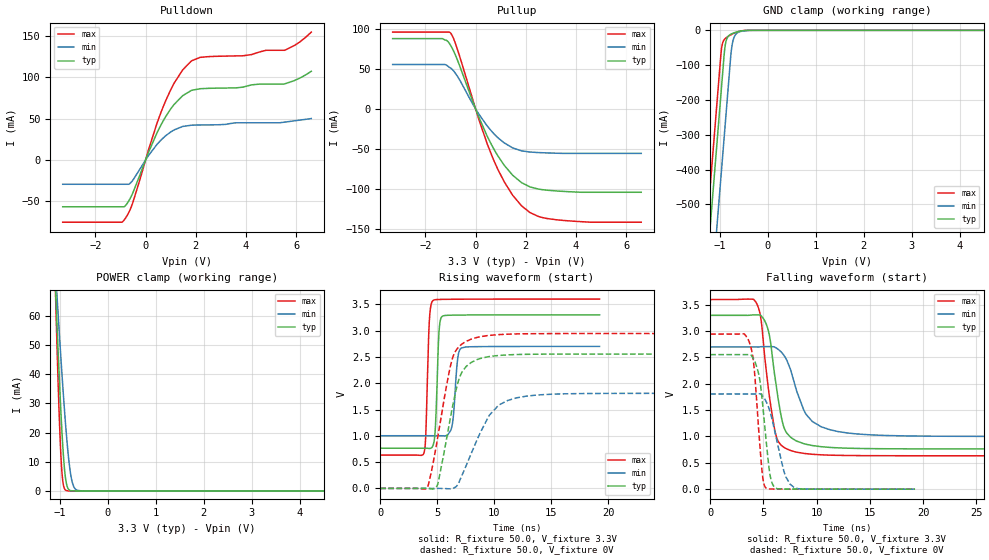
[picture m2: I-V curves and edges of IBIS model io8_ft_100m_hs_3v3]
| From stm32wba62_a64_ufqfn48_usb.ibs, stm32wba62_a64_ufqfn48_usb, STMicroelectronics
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[Model]   io8_ft_100m_hs_3v3
Model_type I/O
Polarity   Non-Inverting
Enable   Active-Low
| CAP_THRESHOLD on pad IOFT is "UDTCAPC" :
| Rising=30.0% of vddiom   Falling=70.0% of vddiom
| C_comp min and max val. don't necessarily correlate with the min and max pvt
| but are the smallest and greatest pad capacitance found.
| var   typ   min   max
C_comp   3.79770pF  3.69238pF  3.85115pF
|C_comp_pullup   2.35247pF  2.17461pF  2.43366pF
|C_comp_pulldown   1.44523pF  1.51776pF  1.41750pF
Vinl = 1.35V
Vinh = 1.8V
Vmeas = 1.65V   | Reference voltage for timing measurements
Cref  = 50.0pF   | Timing specification test load capacitance value
Rref  = 1.0MOhm   | Timing specification test load resistance value
Vref  = 1.815V   | Timing specification test load voltage
[Model Spec]
| TIME_THRESHOLD on pin ZIV11 is "CMOS" :
| Rising=50.0% of vdd   Falling=50.0% of vdd
Vinl 1.29050V 1.08050V 1.37650V
Vinh 1.79850V 1.52050V 1.90250V
| variable   typ   min   max
[Temperature Range] 25.0 140.0 -40.0
| variable   typ   min   max
[Voltage Range] 3.3V 2.7V 3.6V
| variable   typ   min   max
[POWER Clamp Reference] 3.3V 2.7V 3.6V
| variable   typ   min   max
[GND Clamp Reference] 0V 0V 0V
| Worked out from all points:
|   slope of the pulldown table from 0 to 0.495 V, typ, clamps not added: 14 ohm
|   slope of the pullup table from 0 to 0.495 V, typ, clamps not added: 13.8 ohm
|   GND clamp passes 1 mA (typ) near -0.51 V on its own axis
|   POWER clamp passes 1 mA (typ) near -0.83 V on its own axis
|   rising waveform, R_fixture 50.0, V_fixture 3.3V: 20-80 % time 250ps typ, 341ps min, 242ps max; typ from 0.764 V to 3.3 V
|   falling waveform, R_fixture 50.0, V_fixture 3.3V: 20-80 % time 1.12ns typ, 1.98ns min, 1.08ns max; typ from 3.3 V to 0.764 V
|   rising waveform, R_fixture 50.0, V_fixture 0V: 20-80 % time 1.41ns typ, 2.41ns min, 1.46ns max; typ from 0 V to 2.55 V
|   falling waveform, R_fixture 50.0, V_fixture 0V: 20-80 % time 784ps typ, 1.24ns min, 661ps max; typ from 2.55 V to 0 V
[POWER Clamp]
-3.3V     1.123A     753mA      1.645A
-1.09V    69.42mA    75.17mA    67.14mA
-1.08V    65.31mA    72.42mA    61.23mA
-1.06V    57.23mA    66.98mA    49.77mA
-1.01V    38.06mA    53.68mA    24.29mA
-970mV    24.36mA    43.46mA    9.575mA
-930mV    13.06mA    33.74mA    2.352mA
-870mV    3.065mA    20.56mA    165.9uA
-810mV    418.4uA    10.06mA    10.3uA
-760mV    69.41uA    4.321mA    1.009uA
-630mV    611.5nA    197uA      2.727nA
6.6V      0A         0A         0A
[GND Clamp]
-3.3V     -4.134A    -4.372A    -4.018A
-1.59V    -1.227A    -1.465A    -1.111A
-1.25V    -648.9mA   -886.9mA   -533mA
-980mV    -189.9mA   -427.9mA   -74mA
-960mV    -155.9mA   -393.9mA   -48.8mA
-910mV    -70.86mA   -308.9mA   -27.2mA
-880mV    -37.23mA   -257.9mA   -22.76mA
-770mV    -11.28mA   -71.59mA   -12.95mA
-730mV    -8.709mA   -32.74mA   -10.07mA
-630mV    -4.122mA   -6.943mA   -4.354mA
-370mV    -42.68uA   -212.2uA   -13.03uA
6.6V      2.311nA    506.4nA    1.057nA
| variable   typ   min   max
[Pullup Reference] 3.3V 2.7V 3.6V
| variable   typ   min   max
[Pulldown Reference] 0V 0V 0V
[Pullup]
-3.3V     87.39mA    55.15mA    95.56mA
-1.32V    87.39mA    55.15mA    95.56mA
-990mV    78.89mA    50.68mA    94.2mA
-710mV    59.88mA    39.92mA    72.92mA
120mV     -9.566mA   -6.09mA    -12.19mA
460mV     -33.83mA   -21.24mA   -43.26mA
800mV     -54.04mA   -33.36mA   -69.41mA
1.48V     -82.86mA   -48.82mA   -107.8mA
2.17V     -97.42mA   -53.93mA   -129.4mA
2.7V      -101mA     -54.85mA   -135.9mA
3.48V     -102.9mA   -55.62mA   -139.1mA
6.6V      -104.1mA   -55.62mA   -141.4mA
[Pulldown]
-3.3V     -56.7mA    -29.42mA   -75.36mA
-860mV    -56.67mA   -29.42mA   -72.94mA
-520mV    -40.69mA   -25.01mA   -52.64mA
460mV     33.25mA    19.09mA    44.92mA
800mV     52.54mA    29.36mA    71.75mA
1.14V     67.41mA    36.49mA    93.2mA
1.48V     77.97mA    40.67mA    109.3mA
1.83V     84.38mA    42.18mA    120.1mA
2.17V     86.37mA    42.45mA    124.3mA
3.88V     88.31mA    45.1mA     126.3mA
5.54V     92.28mA    45.89mA    133mA
6.6V      107.5mA    50.2mA     155mA
[Ramp]
dV/dt_r 1.53258V/1.41096ns 1.08444V/2.3585ns 1.76673V/1.46232ns
dV/dt_f 1.52157V/1.123ns 1.019V/1.90096ns 1.77971V/1.07619ns
R_load = 50.0
| Removed startup time: 0s 0s 0s  .
| Removed end time: 19.25ns.
[Rising Waveform]
R_fixture   = 50.0
V_fixture   = 3.3V
V_fixture_min = 2.7V
V_fixture_max = 3.6V
0s        764mV      1.002V     633.8mV
3.85ns    764.1mV    1.002V     683.9mV
4ns       764mV      1.002V     1.032V
4.3ns     759.9mV    1.002V     3.154V
4.65ns    825.9mV    1.002V     3.576V
5.15ns    2.948V     1.002V     3.592V
5.4ns     3.265V     1.001V     3.594V
6.3ns     3.294V     1.188V     3.596V
7.1ns     3.296V     2.667V     3.597V
19.25ns   3.3V       2.7V       3.6V
| Removed startup time: 0s 0s 0s  .
| Removed end time: 39.25ns.
[Falling Waveform]
R_fixture   = 50.0
V_fixture   = 3.3V
V_fixture_min = 2.7V
V_fixture_max = 3.6V
0s        3.3V       2.7V       3.6V
4.4ns     3.308V     2.7V       3.512V
4.8ns     3.289V     2.705V     3.187V
5.45ns    3.02V      2.706V     1.939V
6.15ns    2.041V     2.687V     1.047V
6.85ns    1.226V     2.562V     805.4mV
7.55ns    985.9mV    2.273V     734.1mV
9ns       853mV      1.423V     674.2mV
12.05ns   784mV      1.092V     641.9mV
39.25ns   764mV      1.002V     633.8mV
| Removed startup time: 0s 0s 0s  .
| Removed end time: 39.2ns.
[Rising Waveform]
R_fixture   = 50.0
V_fixture   = 0V
V_fixture_min = 0V
V_fixture_max = 0V
0s        20.8nV     123.7nV    58.33nV
4.15ns    -261.4uV   4.517uV    22.09mV
5.05ns    82.9mV     56.07uV    976.1mV
6.3ns     1.503V     -4.527mV   2.444V
7ns       2.13V      160.7mV    2.714V
8ns       2.397V     670.8mV    2.839V
9.5ns     2.505V     1.362V     2.908V
10.4ns    2.528V     1.584V     2.924V
12.8ns    2.549V     1.753V     2.94V
39.2ns    2.554V     1.807V     2.945V
| Removed startup time: 0s 0s 0s  .
| Removed end time: 19.25ns.
[Falling Waveform]
R_fixture   = 50.0
V_fixture   = 0V
V_fixture_min = 0V
V_fixture_max = 0V
0s        2.554V     1.807V     2.945V
3.7ns     2.557V     1.807V     2.777V
4.1ns     2.462V     1.807V     2.361V
4.6ns     2.143V     1.81V      1.009V
4.95ns    1.567V     1.762V     203.2mV
5.25ns    935.7mV    1.665V     19.09mV
5.9ns     79.06mV    1.25V      2.645mV
7ns       2.539mV    292.4mV    1.374mV
7.9ns     1.543mV    29.69mV    1.011mV
19.25ns   28.11uV    81.24uV    25uV
